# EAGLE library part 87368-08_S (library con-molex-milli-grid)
RECEPTACAL
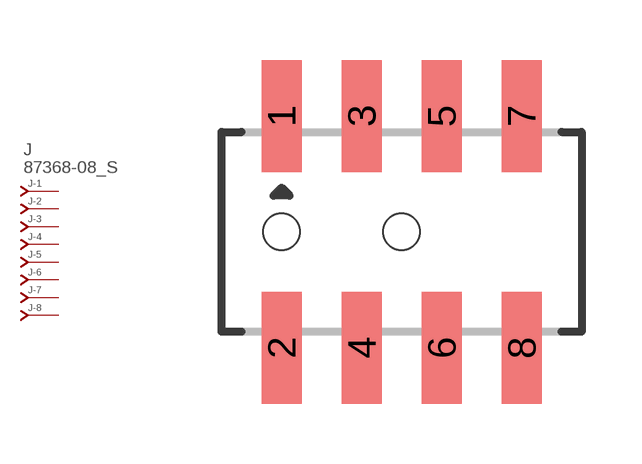
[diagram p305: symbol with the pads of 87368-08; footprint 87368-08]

Designator prefix J; gates -1=J-NV -2=J-N -3=J-N -4=J-N -5=J-N -6=J-N -7=J-N -8=J-N

## 87368-08_S  [87368-08]
1  -1:J  pas
2  -2:J  pas
3  -3:J  pas
4  -4:J  pas
5  -5:J  pas
6  -6:J  pas
7  -7:J  pas
8  -8:J  pas

## Footprint 87368-08 (pad centres in mm)
RECEPTACAL Dual Row, Side Entry
smd 1 x 2.8: 1 -3,2.9; 2 -3,-2.9; 3 -1,2.9; 4 -1,-2.9; 5 1,2.9; 6 1,-2.9; 7 3,2.9; 8 3,-2.9
hole 0.914 at -3,0
hole 0.914 at 0,0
